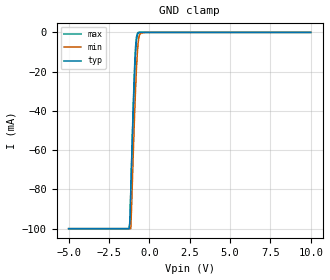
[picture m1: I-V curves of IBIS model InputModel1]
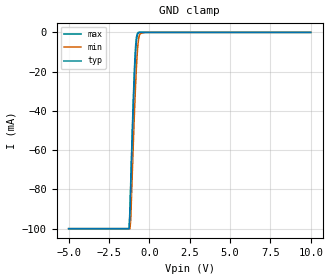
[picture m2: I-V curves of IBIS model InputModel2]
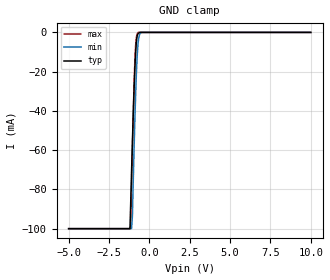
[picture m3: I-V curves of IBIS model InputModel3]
[IBIS Ver]   2.1
[File name]   e_002bc5.ibs   | e_= TSOP, f002bc= abbr chip name, 5 = 5V Vcc
[File Rev]   2.00
[Date]   3-April-96
[Source]   File generated from lab measurements at Intel Corporation
[Notes]   This model is for both the 28F002BC-T & 28F002BC-B.
   Rev 2.00 All data was replaced by actual measurements
   performed in a lab.
[Disclaimer] INTEL DEVELOPER'S SOFTWARE LICENSE AGREEMENT
| BY USING THIS SOFTWARE, YOU ARE AGREEING TO BE BOUND
| BY THE TERMS OFTHIS AGREEMENT.  DO NOT USE THE SOFTWARE
| UNTIL YOU HAVE CAREFULLY READAND AGREED TO THE FOLLOWING
| TERMS AND CONDITIONS.  IF YOU DO NOT AGREETO THE TERMS
| OF THIS AGREEMENT, PROMPTLY RETURN THE SOFTWARE PACKAGE
| ANDANY ACCOMPANYING ITEMS.
| IF YOU USE THIS SOFTWARE, YOU WILL BE BOUND BY THE TERMS
| OF THIS AGREEMENT
| LICENSE: Intel Corporation ("Intel") grants you the non-exclusive right
| to use the enclosed software program ("Software").  You will not use,
| copy, modify, rent, sell or transfer the Software or any portion
| thereof, except as provided in this Agreement.
| System OEM Developers may:
| 1.   Copy the Software for support, backup or archival purposes;
| 2.   Install, use, or distribute Intel owned Software in object code
|   only;
| 3.   Modify and/or use Software source code that Intel directly makes
|   available to you as an OEM Developer;
| 4.   Install, use, modify, distribute, and/or make or have made
|   derivatives ("Derivatives") of Intel owned Software under the
|   terms and conditions in this Agreement, ONLY if you are a System
|   OEM Developer and NOT an end-user.
| RESTRICTIONS:
| YOU WILL NOT:
| 1.   Copy the Software, in whole or in part, except as provided for
|   in this Agreement;
| 2.   Decompile or reverse engineer any Software provided in object
|   code format;
| 3.   Distribute any Software or Derivative code to any end-users,
|   unless approved by Intel in a prior writing.
| TRANSFER: You may transfer the Software to another OEM
| Developer if thereceiving party agrees to the terms of this
| Agreement at the sole risk of any receiving party.
| OWNERSHIP AND COPYRIGHT OF SOFTWARE:
| Title to the Software and all copies thereof remain with Intel
| or its vendors.  The Software iscopyrighted and is protected by
| United States and international copyright laws.  You will not
| remove the copyright notice from the Software.  You agree to
| prevent any unauthorized copying of the Software.
| DERIVATIVE WORK: OEM Developers that make or have made
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[Copyright]   Copyright 1996, Intel Corporation, All Rights Reserved
[Component]   E28F002BC   | 40-lead TSOP package, 28F002BC
[Manufacturer]  Intel   | Boot Block (tm)
|   | operating in 5V Vcc range
[Package]
| The following values apply for the Alloy-42 leadframe.
|Variable   typ   min   max
R_pkg   135m   126m   144m
L_pkg   3.95nH   3.62nH   4.28nH
C_pkg   0.39pF   0.38pF   0.40pF
|***********************Pin Definition********************************
[Pin]   signal_name   model_name   R_pin   L_pin   C_pin
  1   A16   InputModel2
  2   A15   InputModel1
  3   A14   InputModel1
  4   A13   InputModel1
  5   A12   InputModel1
  6   A11   InputModel1
  7   A9   InputModel1
  8   A8   InputModel1
  9   WE#   InputModel3
 10   RP#   InputModel3
 11   VPP   POWER
 12   WP#   InputModel3
 13   NC   InputModel1
 14   A7   InputModel1
 15   A6   InputModel1
 16   A5   InputModel1
 17   A4   InputModel1
 18   A3   InputModel1
 19   A2   InputModel1
 20   A1   InputModel1
 21   A0   InputModel2
 22   CE#   InputModel3
 23   GND   GND
 24   OE#   InputModel3
 25   DQ0   InputOutput
 26   DQ1   InputOutput
 27   DQ2   InputOutput
 28   DQ3   InputOutput
 29   NC   InputModel4
 30   VCC   POWER
 31   VCC   POWER
 32   DQ4   InputOutput
 33   DQ5   InputOutput
 34   DQ6   InputOutput
 35   DQ7   InputOutput
 36   A10   InputModel1
 37   NC   InputModel4
 38   NC   InputModel4
 39   GND   GND
 40   A17   InputModel2
|***********************Input Model 4******************************
[Model]   InputModel4
Model_type   Input
|   Model for  DU & NC pins, excluding Pin #13.
Vinl = 0.8V
Vinh = 2.0V
|Variable   Typ   Min   Max
C_comp   5.61p   NA   7.6p
[Voltage Range]   5.0V   4.5V   5.5V
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| Models and submodels in the file (5): InputModel1 (Input), InputModel2 (Input), InputModel3 (Input), InputModel4 (Input), InputOutput (I/O)
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|*********************Input Model 1************************************
[Model]   InputModel1
Model_type   Input
|   Model for A[8:15] A[1:7] & NC (pin 13).
Vinl = 0.8V
Vinh = 2.0V
|Variable   Typ   Min   Max
C_comp   5.61p   NA   7.6p
[Voltage Range]   5.0V   4.5V   5.5V
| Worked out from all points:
|   GND clamp passes 1 mA (typ) near -0.72 V on its own axis
[GND_clamp]
|Voltage  I(typ)   I(min)   I(max)
-5V       -100mA     -100mA     -100mA
-1.25V    -100mA     -100mA     -100mA
-1.2V     -95.3mA    -100mA     -96.97mA
-1.15V    -80.92mA   -100mA     -81.41mA
-1V       -40.48mA   -62.87mA   -37.82mA
-900mV    -18.21mA   -38.72mA   -14.64mA
-850mV    -10.1mA    -28.28mA   -6.908mA
-800mV    -4.427mA   -18.77mA   -2.472mA
-700mV    -589.5uA   -5.79mA    0A
-600mV    0A         -1.063mA   0A
-250mV    0A         0A         0A
10V       0A         0A         0A
[Power_clamp]
| Input buffer circuits of this product do not intrinsically
| require a [Power_clamp] definition.  This zero current
| [Power_clamp] table is provided for the compatibility with
| some IBIS parsers.
|Voltage  I(typ)   I(min)   I(max)
-5V       0A         0A         0A
0V        0A         0A         0A
5V        0A         0A         0A
10V       0A         0A         0A
|*********************Input Model 2******************************
[Model]   InputModel2
Model_type   Input
|   Model for A[0], A[16] & A[17] pins.
Vinl = 0.8V
Vinh = 2.0V
|Variable   Typ   Min   Max
C_comp   5.61p   NA   7.6p
[Voltage Range]   5.0V   4.5V   5.5V
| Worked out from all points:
|   GND clamp passes 1 mA (typ) near -0.72 V on its own axis
[GND_clamp]
|Voltage  I(typ)   I(min)   I(max)
-5V       -100mA     -100mA     -100mA
-1.25V    -100mA     -100mA     -100mA
-1.2V     -92.25mA   -100mA     -89.48mA
-1.15V    -78.35mA   -95.31mA   -75.23mA
-1V       -39.26mA   -58.42mA   -35.27mA
-900mV    -17.72mA   -36.17mA   -13.9mA
-850mV    -9.851mA   -26.51mA   -6.694mA
-800mV    -4.349mA   -17.72mA   -2.426mA
-700mV    -587.2uA   -5.568mA   0A
-600mV    0A         -1.028mA   0A
-250mV    0A         0A         0A
10V       0A         0A         0A
[Power_clamp]
| Input buffer circuits of this product do not intrinsically
| require a [Power_clamp] definition.  This zero current
| [Power_clamp] table is provided for the compatibility with
| some IBIS parsers.
|Voltage  I(typ)   I(min)   I(max)
-5V       0A         0A         0A
0V        0A         0A         0A
5V        0A         0A         0A
10V       0A         0A         0A
|***********************Input Model 3******************************
[Model]   InputModel3
Model_type   Input
|   Model for WE#, WP#, RP#, OE# & CE# pin.
Vinl = 0.8V
Vinh = 2.0V
|Variable   Typ   Min   Max
C_comp   5.61p   NA   7.6p
[Voltage Range]   5.0V   4.5V   5.5V
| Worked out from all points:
|   GND clamp passes 1 mA (typ) near -0.72 V on its own axis
[GND_clamp]
|Voltage  I(typ)   I(min)   I(max)
-5V       -100mA     -100mA     -100mA
-1.2V     -100mA     -100mA     -100mA
-1.15V    -85.5mA    -100mA     -98.31mA
-1.1V     -70.41mA   -100mA     -78.56mA
-1.05V    -56.02mA   -93.54mA   -59.94mA
-950mV    -29.73mA   -60.51mA   -27.3mA
-900mV    -18.71mA   -45.27mA   -14.84mA
-850mV    -10.25mA   -31.97mA   -6.48mA
-800mV    -4.452mA   -20.32mA   -2.166mA
-700mV    -580.8uA   -5.673mA   0A
-500mV    0A         0A         0A
10V       0A         0A         0A
[Power_clamp]
| Input buffer circuits of this product do not intrinsically
| require a [Power_clamp] definition.  This zero current
| [Power_clamp] table is provided for the compatibility with
| some IBIS parsers.
|Voltage  I(typ)   I(min)   I(max)
-5V       0A         0A         0A
0V        0A         0A         0A
5V        0A         0A         0A
10V       0A         0A         0A
